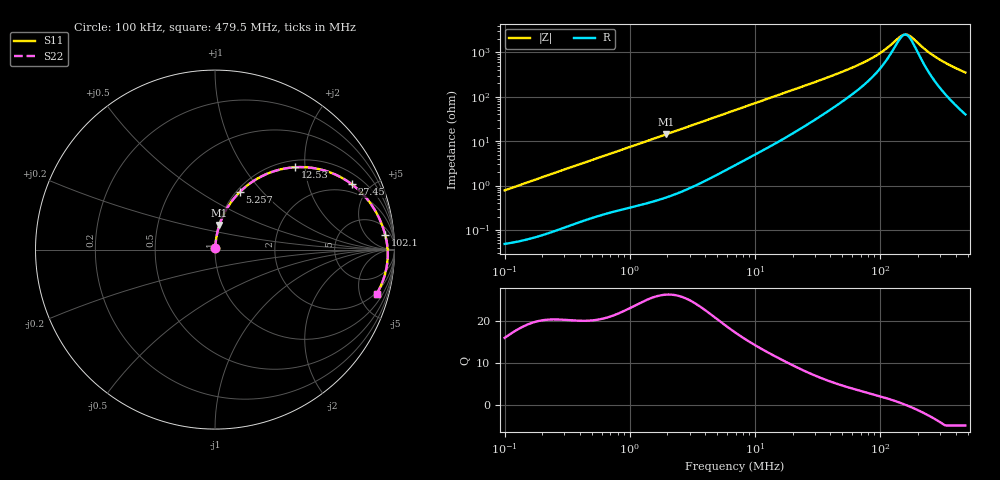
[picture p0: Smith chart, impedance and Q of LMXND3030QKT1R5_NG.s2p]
! LMXND3030QKT1R5_NG  S-PARAMETER MODEL  ( General Type )
! Model Generated by TAIYO YUDEN Corporation (https://www.yuden.co.jp/en/)
! Version 1.0
! TAIYO YUDEN Control No. 191023NI43SB-FBB
! Copyright(c) 2019 TAIYO YUDEN CO.,LTD. All Rights Reserved.
! Product Description (link to TY-COMPAS)
! https://ds.yuden.co.jp/TYCOMPAS/or/detail?pn=LMXND3030QKT1R5NNG&u=M
! Products Name : Inductors
! Characteristics :
!  Inductance : 1.5 uH , SRF(min) : 87 MHz , DC Resistance(max) : 0.0456 Ohm
!  Rated Current : Saturation :1800 mA , Temp Rise : 1820 mA (40 degC)
!  Case Size : 3.0 x 3.0 / 0.118 x 0.118 [mm/inch] , Thickness : 1.5 / 0.059 [mm/inch]
!  (Conditions: Temperature = 25 degC , DC Bias Current/Voltage = 0A / 0V)
! External Node Assignments :
!  1  o---GGG---o  2
! GND o---------o GND
! Frequency Range : 0.1MHz  -  479.524407MHz  [ 402 STEP ]
# MHz S RI R 50
! Freq[MHz].  S11 Real  S11 Imag  S21 Real  S21 Imag  S12 Real  S12 Imag  S22 Real  S22 Imag
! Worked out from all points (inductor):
!   401 points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, 100 kHz to 479.5 MHz, reference 50 ohm
!   read as one part in series: L = 1.23 uH near 104.3 kHz
!   highest Q = 26.4 at 1.942 MHz (marker M1), where L = 1.16 uH
!   self-resonance near 157.7 MHz
!   S11 on the Smith chart (normalised r, x): 100 kHz: 1.00, +0.02; 5.257 MHz: 1.04, +0.76; 12.53 MHz: 1.14, +1.77; 27.45 MHz: 1.51, +3.85; 102.1 MHz: 10, +18; 479.5 MHz: 1.80, -6.96
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0.1  0.000546 0.00776  0.9995 -0.00776  0.9995 -0.00776  0.000546 0.00776
0.413557  0.00254 0.0312  0.9975 -0.0312  0.9975 -0.0312  0.00254 0.0312
1.710297  0.0199 0.1217  0.9801 -0.1217  0.9801 -0.1217  0.0199 0.1217
1.942154  0.0246 0.1372  0.9754 -0.1372  0.9754 -0.1372  0.0246 0.1372
3.369275  0.0645 0.2258  0.9355 -0.2258  0.9355 -0.2258  0.0645 0.2258
5.257497  0.1372 0.3199  0.8628 -0.3199  0.8628 -0.3199  0.1372 0.3199
7.073061  0.2172 0.3842  0.7828 -0.3842  0.7828 -0.3842  0.2172 0.3842
12.5332  0.4447 0.4588  0.5553 -0.4588  0.5553 -0.4588  0.4447 0.4588
17.96787  0.6059 0.4418  0.3941 -0.4418  0.3941 -0.4418  0.6059 0.4418
27.44967  0.7618 0.3644  0.2382 -0.3644  0.2382 -0.3644  0.7618 0.3644
28.6379  0.7743 0.3548  0.2257 -0.3548  0.2257 -0.3548  0.7743 0.3548
41.0559  0.8574 0.2692  0.1426 -0.2692  0.1426 -0.2692  0.8574 0.2692
61.40647  0.9124 0.1793  0.0876 -0.1793  0.0876 -0.1793  0.9124 0.1793
80.87987  0.9355 0.1241  0.0645 -0.1241  0.0645 -0.1241  0.9355 0.1241
102.1087  0.9489 0.0802  0.0511 -0.0802  0.0511 -0.0802  0.9489 0.0802
118.4342  0.955 0.0529  0.045 -0.0529  0.045 -0.0529  0.955 0.0529
146.3852  0.9606 0.0139  0.0394 -0.0139  0.0394 -0.0139  0.9606 0.0139
155.9923  0.9616 0.00206  0.0384 -0.00206  0.0384 -0.00206  0.9616 0.00206
166.23  0.9623 -0.00991  0.0377 0.00991  0.0377 0.00991  0.9623 -0.00991
276.4127  0.9532 -0.1128  0.0468 0.1128  0.0468 0.1128  0.9532 -0.1128
364.0696  0.9344 -0.1767  0.0656 0.1767  0.0656 0.1767  0.9344 -0.1767
479.5244  0.9007 -0.2473  0.0993 0.2473  0.0993 0.2473  0.9007 -0.2473
